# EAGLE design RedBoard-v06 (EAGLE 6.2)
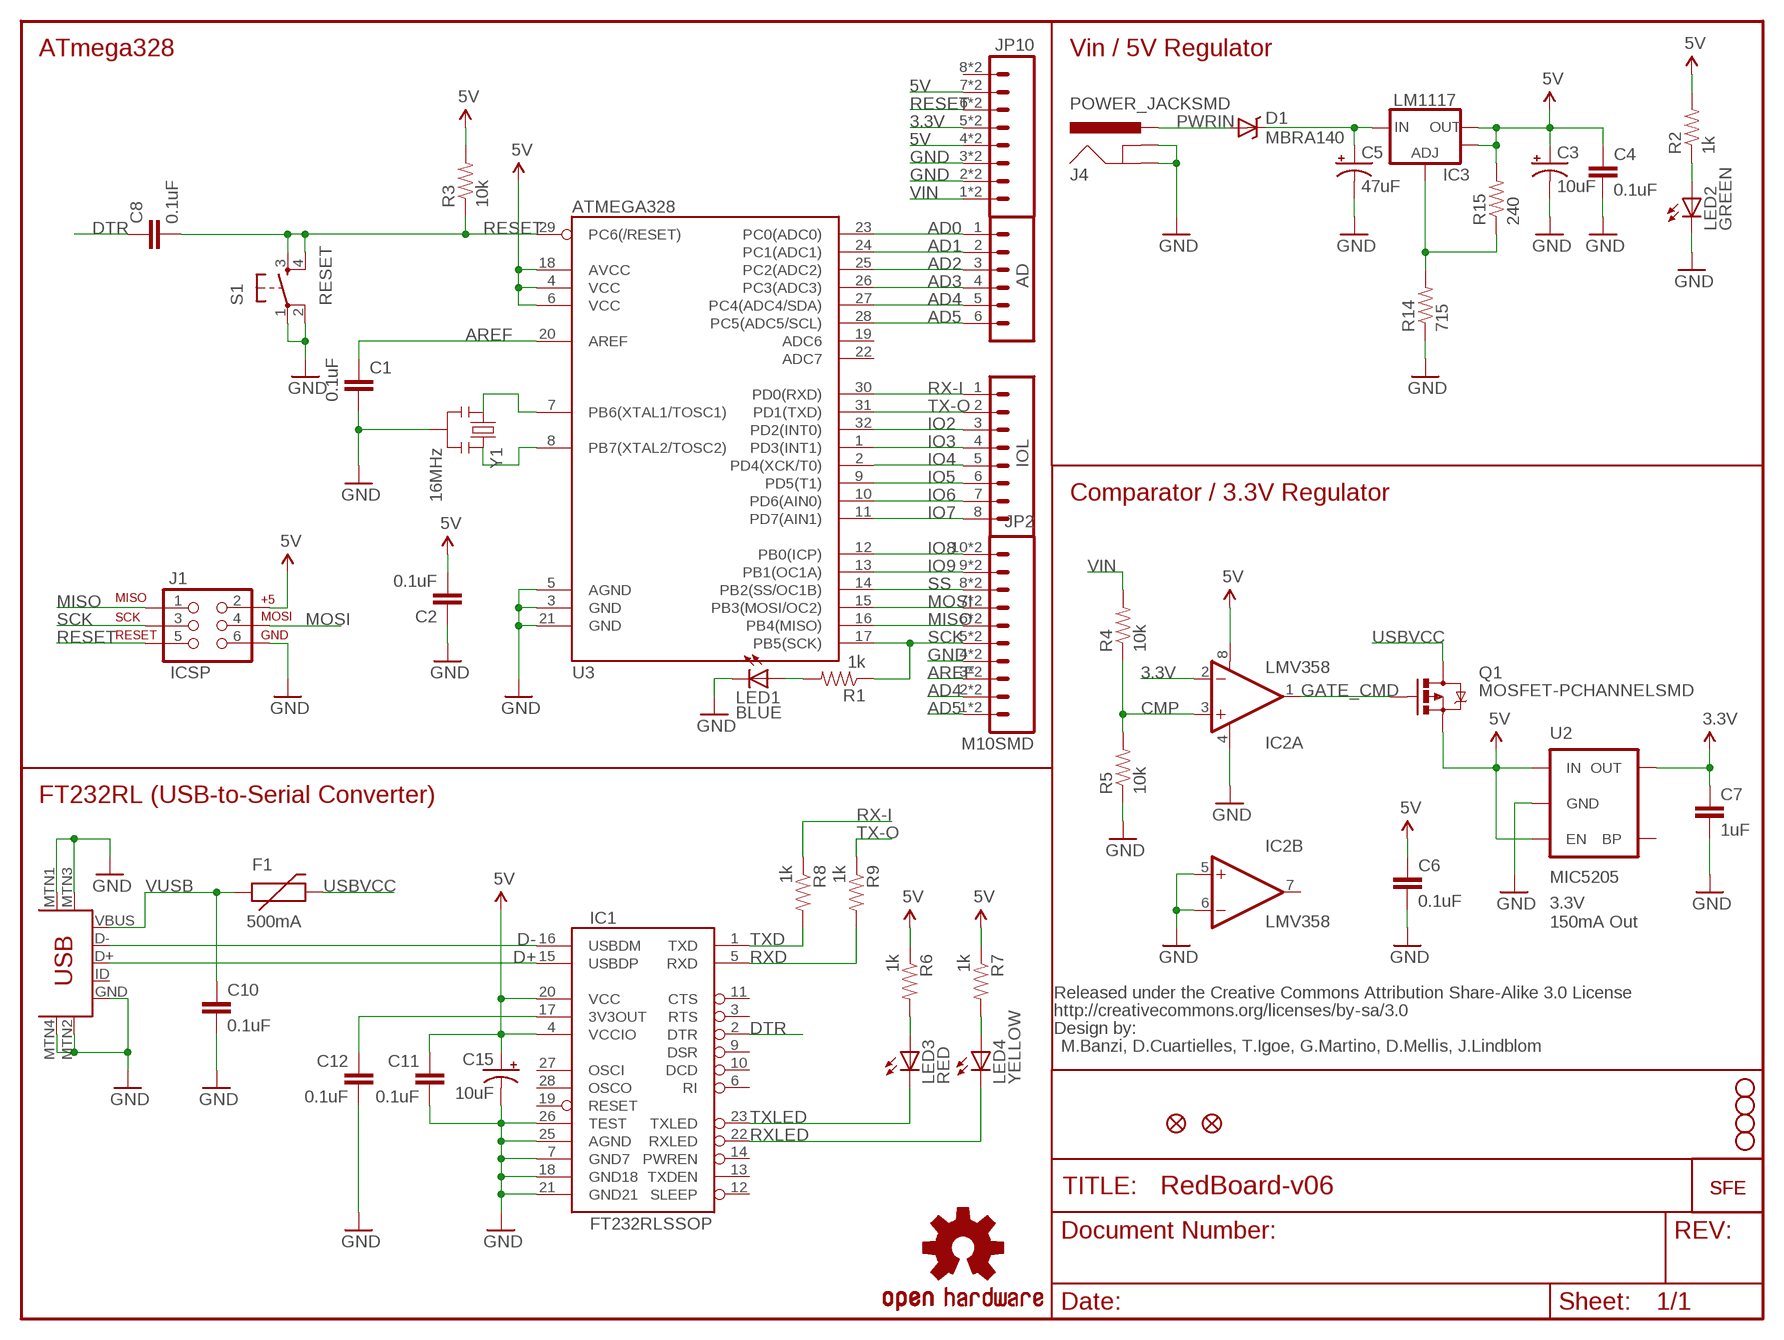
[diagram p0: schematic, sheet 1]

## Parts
AD  M06SMD-STRAIGHT-COMBO  [1X06_SMD_STRAIGHT_COMBO]
C1  0.1uF  CAP0402-CAP  [0402-CAP]
C2  0.1uF  CAP0402-CAP  [0402-CAP]
C3  10uF  CAP_POL1206  [EIA3216]
C4  0.1uF  CAP0402-CAP  [0402-CAP]
C5  47uF  CAP_POLD  [PANASONIC_D]
C6  0.1uF  CAP0402-CAP  [0402-CAP]
C7  1uF  CAP0402-CAP  [0402-CAP]
C8  0.1uF  CAP0402-CAP  [0402-CAP]
C10  0.1uF  CAP0402-CAP  [0402-CAP]
C11  0.1uF  CAP0402-CAP  [0402-CAP]
C12  0.1uF  CAP0402-CAP  [0402-CAP]
C15  10uF  CAP_POL1206  [EIA3216]
D1  MBRA140  DIODE-SCHOTTKY_  [SMA-DIODE]
F1  500mA  PTCSMD  [PTC-1206]
IC1  FT232RLSSOP  [SSOP28DB]
IC2  LMV358  OPAMP-DUALU  [SO08]
IC3  LM1117  V_REG_LM1117ALT1  [SOT223-ALT1]
IOL  M08SMD-COMBO  [1X08_SMD_COMBINED]
J1  ICSP  AVR_SPI_PRG_6PTH  [2X3]
J4  POWER_JACKSMD  [POWER_JACK_SMD]
JP1  LOGO-SFENW2  [SFE-NEW-WEB]
JP2  M10SMD  [1X10_SMD_COMBINED]
JP3  STAND-OFF  [STAND-OFF]
JP4  STAND-OFF  [STAND-OFF]
JP5  STAND-OFF  [STAND-OFF]
JP6  STAND-OFF  [STAND-OFF]
JP7  LOGO-SFESK  [SFE-LOGO-FLAME]
JP8  FIDUCIAL1X2  [FIDUCIAL-1X2]
JP9  FIDUCIAL1X2  [FIDUCIAL-1X2]
JP10  M08SMD-COMBO  [1X08_SMD_COMBINED]
LED1  BLUE  LED0603  [LED-0603]
LED2  GREEN  LED0603  [LED-0603]
LED3  RED  LED0603  [LED-0603]
LED4  YELLOW  LED0603  [LED-0603]
Q1  MOSFET-PCHANNELSMD  [SOT23-3]
R1  1k  RESISTOR0402-RES  [0402-RES]
R2  1k  RESISTOR0402-RES  [0402-RES]
R3  10k  RESISTOR0402-RES  [0402-RES]
R4  10k  RESISTOR0402-RES  [0402-RES]
R5  10k  RESISTOR0402-RES  [0402-RES]
R6  1k  RESISTOR0402-RES  [0402-RES]
R7  1k  RESISTOR0402-RES  [0402-RES]
R8  1k  RESISTOR0402-RES  [0402-RES]
R9  1k  RESISTOR0402-RES  [0402-RES]
R14  715  RESISTOR0402-RES  [0402-RES]
R15  240  RESISTOR0402-RES  [0402-RES]
S1  RESET  TAC_SWITCHSMD  [TACTILE_SWITCH_SMD]
U2  MIC5205  V_REG_LDOSMD  [SOT23-5]
U3  ATMEGA328  ATMEGA168  [TQFP32-08]
U$13  USB-MINIB-5PIN  [USB-MINIB]
U$15  CREATIVE_COMMONS  [CREATIVE_COMMONS]
U$16  OSHW-LOGOS  [OSHW-LOGO-S]
Y1  16MHz  RESONATORSMD  [RESONATOR-SMD]

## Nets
3.3V: C7.1 IC2.2(A:-IN) JP10.5 JP10.5@2 U2.5(OUT)
5V: C2.2 C3.A(+) C4.1 C6.1 C11.1 C15.A(+) IC1.4(VCCIO) IC1.20(VCC) IC2.8(A:V+) IC3.2(OUT) IC3.4(OUT) J1.2 JP10.4 JP10.4@2 JP10.7 JP10.7@2 Q1.2(S) R2.2 R3.2 R6.1 R7.1 R15.2 U2.1(IN) U2.3(EN) U3.4(VCC) U3.6(VCC) U3.18(AVCC)
AD0: AD.1 U3.23(PC0(ADC0))
AD1: AD.2 U3.24(PC1(ADC1))
AD2: AD.3 U3.25(PC2(ADC2))
AD3: AD.4 U3.26(PC3(ADC3))
AD4: AD.5 JP2.2 JP2.2@2 U3.27(PC4(ADC4/SDA))
AD5: AD.6 JP2.1 JP2.1@2 U3.28(PC5(ADC5/SCL))
AREF: C1.1 JP2.3 JP2.3@2 U3.20(AREF)
CMP: IC2.3(A:+IN) R4.1 R5.2
D+: IC1.15(USBDP) U$13.D+
D-: IC1.16(USBDM) U$13.D-
DTR: C8.1 IC1.2(DTR)
GATE_CMD: IC2.1(A:OUT) Q1.1(G)
GND: C1.2 C2.1 C3.C(-) C4.2 C5.- C6.2 C7.2 C10.2 C11.2 C12.2 C15.C(-) IC1.7(GND7) IC1.18(GND18) IC1.21(GND21) IC1.25(AGND) IC1.26(TEST) IC2.4(A:V-) IC2.5(B:+IN) IC2.6(B:-IN) J1.6 J4.GND(GNDBREAK) J4.P$4(GND) JP2.4 JP2.4@2 JP10.2 JP10.2@2 JP10.3 JP10.3@2 LED1.C LED2.C R5.1 R14.1 S1.1 S1.2 U2.2(GND) U3.3(GND) U3.5(AGND) U3.21(GND) U$13.GND U$13.MTN1(MTN2) U$13.MTN2(MTN3) U$13.MTN3(MTN1) U$13.MTN4 Y1.2
IO2: IOL.3 U3.32(PD2(INT0))
IO3: IOL.4 U3.1(PD3(INT1))
IO4: IOL.5 U3.2(PD4(XCK/T0))
IO5: IOL.6 U3.9(PD5(T1))
IO6: IOL.7 U3.10(PD6(AIN0))
IO7: IOL.8 U3.11(PD7(AIN1))
IO8: JP2.10 JP2.10@2 U3.12(PB0(ICP))
IO9: JP2.9 JP2.9@2 U3.13(PB1(OC1A))
MISO: J1.1 JP2.6 JP2.6@2 U3.16(PB4(MISO))
MOSI: J1.4 JP2.7 JP2.7@2 U3.15(PB3(MOSI/OC2))
N$1: LED1.A R1.2
N$2: LED2.A R2.1
N$3: U3.7(PB6(XTAL1/TOSC1)) Y1.1
N$4: U3.8(PB7(XTAL2/TOSC2)) Y1.3
N$5: C12.1 IC1.17(3V3OUT)
N$8: LED3.A R6.2
N$10: LED4.A R7.2
N$15: IC3.1(ADJ) R14.2 R15.1
PWRIN: D1.A J4.VIN0(PWR)
RESET: C8.2 J1.5 JP10.6 JP10.6@2 R3.1 S1.3 S1.4 U3.29(PC6(/RESET))
RX-I: IOL.1 R8.1 U3.30(PD0(RXD))
RXD: IC1.5(RXD) R9.2
RXLED: IC1.22(RXLED) LED4.C
SCK: J1.3 JP2.5 JP2.5@2 R1.1 U3.17(PB5(SCK))
SS: JP2.8 JP2.8@2 U3.14(PB2(SS/OC1B))
TX-O: IOL.2 R9.1 U3.31(PD1(TXD))
TXD: IC1.1(TXD) R8.2
TXLED: IC1.23(TXLED) LED3.C
USBVCC: F1.2 Q1.3(D)
VIN: C5.+ D1.C IC3.3(IN) JP10.1 JP10.1@2 R4.2
VUSB: C10.1 F1.1 U$13.VBUS
Unconnected: IC1.3(RTS) IC1.6(RI) IC1.9(DSR) IC1.10(DCD) IC1.11(CTS) IC1.12(SLEEP) IC1.13(TXDEN) IC1.14(PWREN) IC1.19(RESET) IC1.27(OSCI) IC1.28(OSCO) IC2.7(B:OUT) JP10.8 JP10.8@2 U2.4(BP) U3.19(ADC6) U3.22(ADC7) U$13.ID

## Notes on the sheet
- ATmega328 | Vin / 5V Regulator
- Comparator / 3.3V Regulator
- FT232RL (USB-to-Serial Converter)
- 3.3V
  150mA Out
- M.Banzi, D.Cuartielles, T.Igoe, G.Martino, D.Mellis, J.Lindblom

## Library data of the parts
AD = SparkFun:M06: Header 6 Standard 6-pin 0.1" header. Use with straight break away headers (SKU : PRT-00116), right angle break away headers (PRT-00553), swiss pins (PRT-00743), machine pins (PRT-00117), and female headers (PRT-00115). Molex polarized connector foot print use with SKU : PRT-08094 with associated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
C1 C2 C4 C6-C8 C10 C12 = SparkFun:CAP: Capacitor
C3 C5 = SparkFun:CAP_POL: Capacitor Polarized
C11 = SparkFun-Capacitors:CAP: Capacitor
C15 = SparkFun-Capacitors:CAP_POL: Capacitor Polarized
D1 = SparkFun:DIODE-SCHOTTKY
F1 = SparkFun:PTC: Resettable Fuse PTC
IC1 = SparkFun-DigitalIC:FT232RL: USB UART FT232RL 4th Generation USB UART (USB <-> Serial) Controller. Spark Fun Electronics SKU : COM-00650
IC2 = SparkFun:OPAMP-DUAL: Operational Amplifier
IC3 = Testing:V_REG_LM1117: Voltage Regulator LM1117 Standard adjustable voltage regulator but in SMD form. Spark Fun Electronics SKU : COM-00595
IOL = SparkFun:M08: Header 8 Standard 8-pin 0.1" header. Use with straight break away headers (SKU : PRT-00116), right angle break away headers (PRT-00553), swiss pins (PRT-00743), machine pins (PRT-00117), and female headers (PRT-00115).
J1 = SparkFun:AVR_SPI_PRG_6: AVR ISP 6 Pin This is the reduced ISP connector for AVR programming. Common on Arduino. This footprint will take up less PCB space and can be used with a 10-pin to 6-pin adapter such as SKU: BOB-08508
J4 = SparkFun:POWER_JACK: Power Jack This is the standard 5.5mm barrel jack for power. The PTH is the most common, proven, reliable, footprint. All others are experimental. The Slot footprint only works if the mill layer is transmitted to the PCB fab house so be warned. Spark Fun Electronics SKU : PRT-00119. Mating wall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
JP1 JP7 = SparkFun-Aesthetics:LOGO-SFE: Spark Fun Electronics PCB Logo
JP2 = SparkFun-Connectors:M10: Header 10 Standard 10-pin 0.1" header. Use with straight break away headers (SKU : PRT-00116), right angle break away headers (PRT-00553), swiss pins (PRT-00743), machine pins (PRT-00117), and female headers (PRT-00115).
JP3-JP6 = SparkFun:STAND-OFF: Stand Off
JP8 JP9 = SparkFun:FIDUCIAL: Fiducial Alignment Points
JP10 = SparkFun-Connectors:M08: Header 8 Standard 8-pin 0.1" header. Use with straight break away headers (SKU : PRT-00116), right angle break away headers (PRT-00553), swiss pins (PRT-00743), machine pins (PRT-00117), and female headers (PRT-00115).
LED1-LED4 = SparkFun:LED: LEDs
Q1 = SparkFun:MOSFET-PCHANNEL
R1-R9 R14 R15 = SparkFun:RESISTOR: Resistor
S1 = SparkFun:TAC_SWITCH: Momentary Switch Button commonly used for reset or general input. Spark Fun Electronics SKU : COM-00097
U2 = SparkFun:V_REG_LDO: Voltage Regulator LDO Standard 150mA LDO voltage regulator in SOT-23 layout. Micrel part MIC5205. BP (by-pass) pin is used to lower output noise with 470pF cap.
U3 = SparkFun:ATMEGA168
U$13 = SparkFun-Connectors:USB-MINIB: Mini-USB "B" connector with 5th pin broken out. Created new symbol breaking out 5th "ID" pin in mini/micro USB connector spec. See: http://en.wikipedia.org/wiki/Mini_usb#Cables. Uses same footprint as 4-pin symbol. Also added pins to connect to mounting / shield pads if required (probably not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
U$15 = SparkFun:CREATIVE_COMMONS
U$16 = SparkFun-Aesthetics:OSHW-LOGO: Open Source Hardware Logo This logo indicates the piece of hardware it is found on incorporates a OSHW license and/or adheres to the definition of open source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
Y1 = SparkFun-FreqCtrl:RESONATOR: Resonator Small SMD resonator. This is the itty bitty 10/20MHz resonators with built in caps. CSTCE10M0G55 and CSTCE20M0V53. Footprint has been reviewed closely but hasn't been tested yet.

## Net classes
0 default: width 0.152 mm, drill 0.305 mm, clearance 0.152 mm

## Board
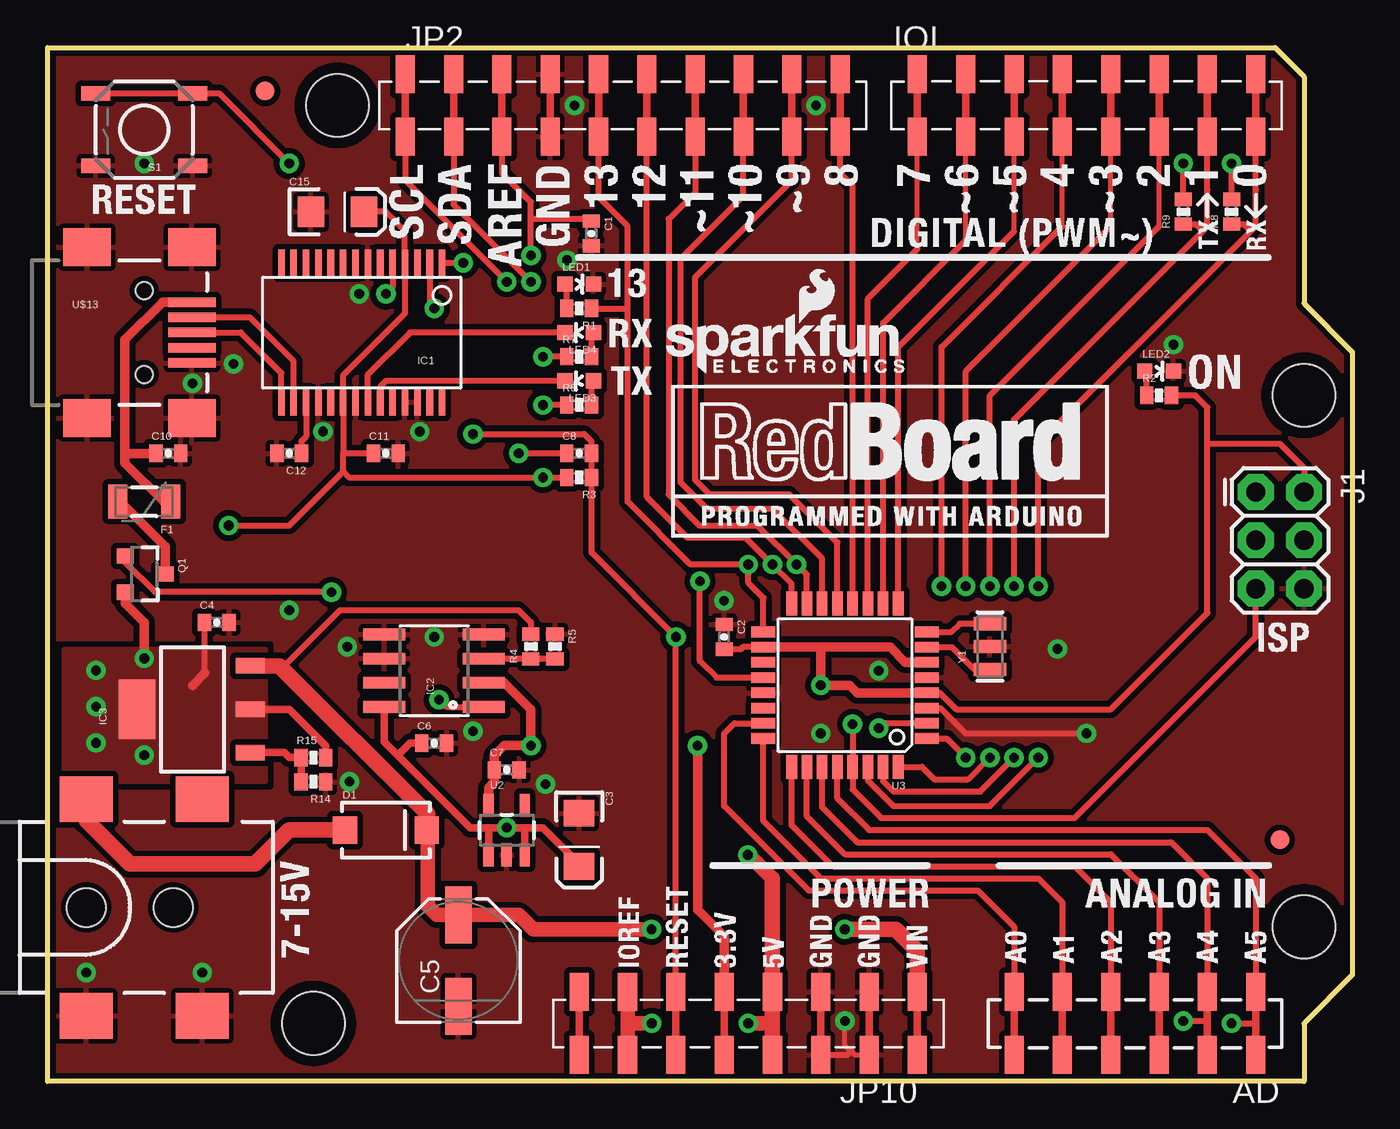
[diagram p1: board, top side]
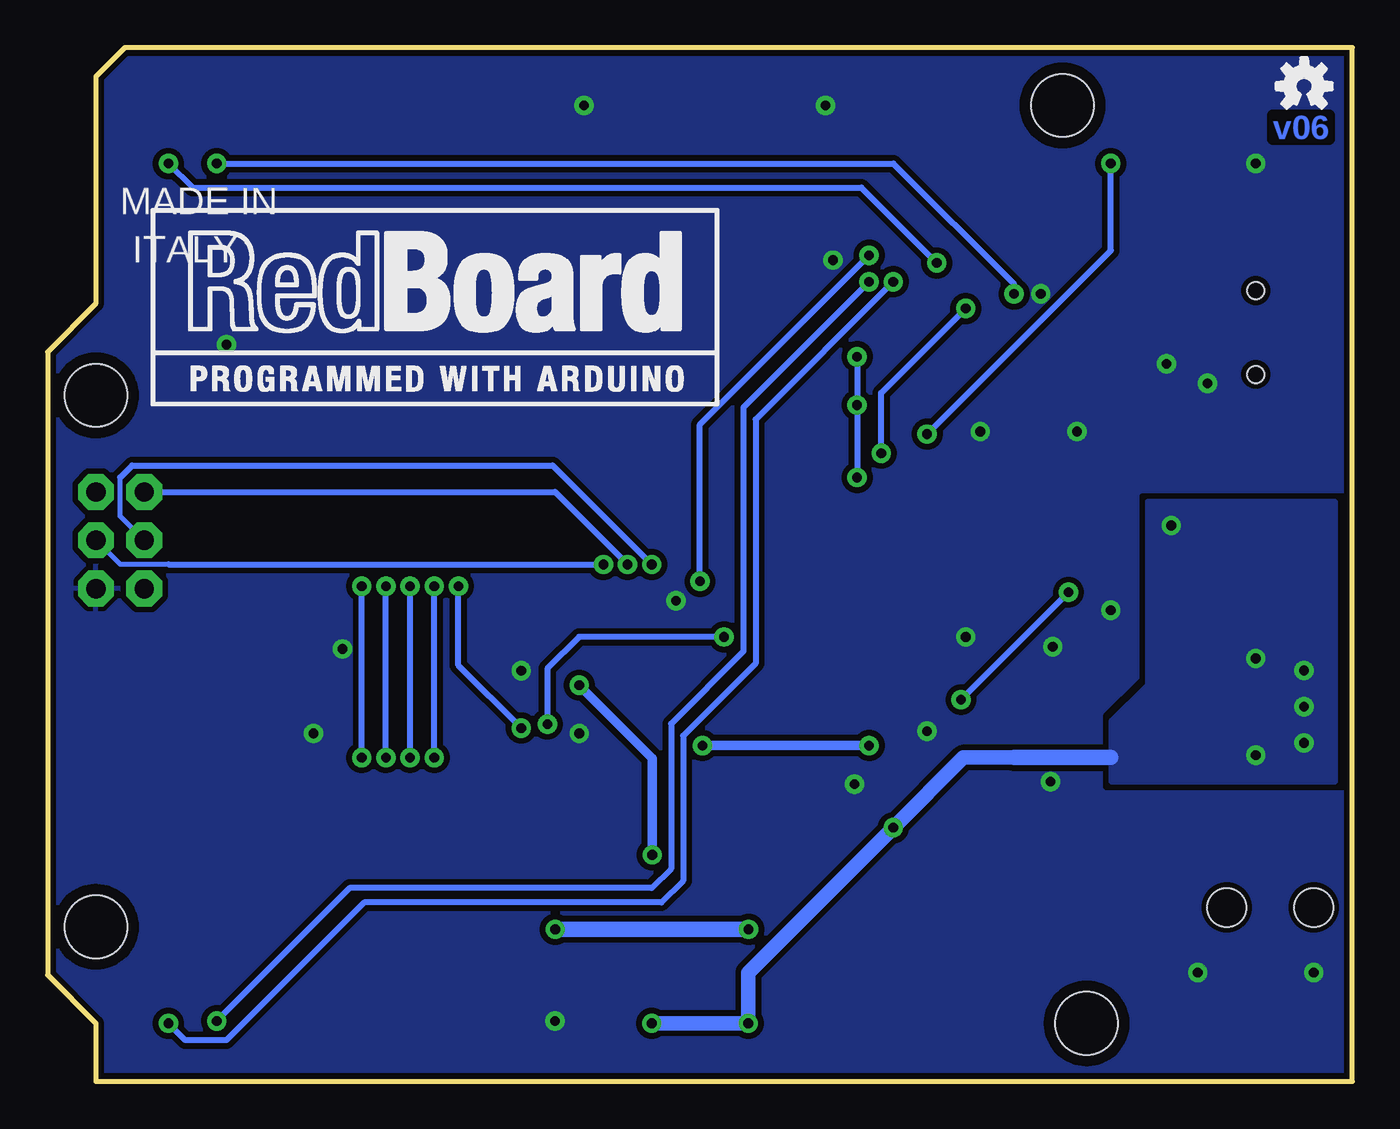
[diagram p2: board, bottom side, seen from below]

Size 68.58 x 54.36 mm. Coordinates in mm from the lower left corner, seen from the top.
Outline: 0,54.36 64.52,54.36 66.04,52.83 66.04,40.89 68.58,38.35 68.58,5.59 66.04,3.05 66.04,0 0,0 0,54.36
Copper layers (1*16): Top 0.035mm / dielectric 1.5mm / Bottom 0.035mm
Design rules: minimum track width 8mil, minimum drill 20mil, track to track 8mil, track to pad 8mil, pad to pad 8mil, via to via 8mil, smd to smd 8mil, copper to edge 8mil, drill to drill 8mil, minimum pad ring 12mil, minimum via ring 10mil, stop-mask expansion 4mil, vias tented up to drill 20mil, thermal gap 10mil
vRestrict: area 0.6,22.4 to 2,30.6; area 5.7,23.1 to 7.4,30.6; area 47.9,10.8 to 48.5,11.3; area 50.4,10.7 to 50.9,11.6; area 11.3,29.3 to 12.7,31.6; area 0.3,13 to 9.4,25

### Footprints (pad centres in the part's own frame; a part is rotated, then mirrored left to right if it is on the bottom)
1X06_SMD_STRAIGHT_COMBO = smd 1 x 2: 1 0,1.65; 1-2 0,-1.65; 2 -2.54,-1.65; 2-2 -2.54,1.65; 3 -5.08,1.65; 3-2 -5.08,-1.65; 4 -7.62,-1.65; 4-2 -7.62,1.65; 5 -10.16,1.65; 5-2 -10.16,-1.65; 6 -12.7,-1.65; 6-2 -12.7,1.65
0402-CAP = smd 0.7 x 0.9: 1 -0.65,0; 2 0.65,0
EIA3216 = smd 1.4 x 1.6: A 1.4,0; C -1.4,0
PANASONIC_D = smd 3 x 1.4: + 2.4,0; - -2.4,0
SMA-DIODE = smd 1.27 x 1.47: A -2.15,0; C 2.15,0
PTC-1206 = smd 1 x 1.8: 1 -1.4,0; 2 1.4,0
SSOP28DB = smd 0.348 x 1.397: 1 -4.225,-3.656; 2 -3.575,-3.656; 3 -2.925,-3.656; 4 -2.275,-3.656; 5 -1.625,-3.656; 6 -0.975,-3.656; 7 -0.325,-3.656; 8 0.325,-3.656; 9 0.975,-3.656; 10 1.625,-3.656; 11 2.275,-3.656; 12 2.925,-3.656; 13 3.575,-3.656; 14 4.225,-3.656; 15 4.225,3.656; 16 3.575,3.656; 17 2.925,3.656; 18 2.275,3.656; 19 1.625,3.656; 20 0.975,3.656; 21 0.325,3.656; 22 -0.325,3.656; 23 -0.975,3.656; 24 -1.625,3.656; 25 -2.275,3.656; 26 -2.925,3.656; 27 -3.575,3.656; 28 -4.225,3.656
SO08 = smd 0.61 x 2.21: 1 -1.905,-2.616; 2 -0.635,-2.616; 3 0.635,-2.616; 4 1.905,-2.616; 5 1.905,2.616; 6 0.635,2.616; 7 -0.635,2.616; 8 -1.905,2.616
SOT223-ALT1 = smd 0.813 x 1.524: 1 -2.271,-3.02; 2 0,-3.02; 3 2.288,-3.02 | smd 3.124 x 1.905: 4 0,2.921
1X08_SMD_COMBINED = smd 1 x 2: 1 0,-1.65; 1@2 0,1.65; 2 -2.54,1.65; 2@2 -2.54,-1.65; 3 -5.08,-1.65; 3@2 -5.08,1.65; 4 -7.62,1.65; 4@2 -7.62,-1.65; 5 -10.16,-1.65; 5@2 -10.16,1.65; 6 -12.7,1.65; 6@2 -12.7,-1.65; 7 -15.24,-1.65; 7@2 -15.24,1.65; 8 -17.78,1.65; 8@2 -17.78,-1.65
2X3 = drill 1.016 pad 1.88 octagon: 1 0,0; 2 0,2.54; 3 2.54,0; 4 2.54,2.54; 5 5.08,0; 6 5.08,2.54
POWER_JACK_SMD = smd 2.8 x 2.4: GND 0,-5.7; P$4 6.1,-5.7; VIN0 0,5.7; VIN1 6.1,5.7 | hole 2.032: 0,0; 4.572,0
1X10_SMD_COMBINED = smd 1 x 2: 1 0,1.65; 1@2 0,-1.65; 2 2.54,-1.65; 2@2 2.54,1.65; 3 5.08,1.65; 3@2 5.08,-1.65; 4 7.62,-1.65; 4@2 7.62,1.65; 5 10.16,1.65; 5@2 10.16,-1.65; 6 12.7,-1.65; 6@2 12.7,1.65; 7 15.24,1.65; 7@2 15.24,-1.65; 8 17.78,-1.65; 8@2 17.78,1.65; 9 20.32,1.65; 9@2 20.32,-1.65; 10 22.86,-1.65; 10@2 22.86,1.65
STAND-OFF = hole 3.302: 0,0
FIDUCIAL-1X2 = smd 1 x 1: 1 0,0
1X08_SMD_COMBINED' = smd 1 x 2: 1 0,1.65; 1@2 0,-1.65; 2 2.54,-1.65; 2@2 2.54,1.65; 3 5.08,1.65; 3@2 5.08,-1.65; 4 7.62,-1.65; 4@2 7.62,1.65; 5 10.16,1.65; 5@2 10.16,-1.65; 6 12.7,-1.65; 6@2 12.7,1.65; 7 15.24,1.65; 7@2 15.24,-1.65; 8 17.78,-1.65; 8@2 17.78,1.65
LED-0603 = smd 0.8 x 0.8: A 0,-0.75; C 0,0.75
SOT23-3 = smd 0.8 x 0.9: 1 -0.95,-1; 2 0.95,-1; 3 0,1.1
0402-RES = smd 0.7 x 0.9: 1 -0.65,0; 2 0.65,0
TACTILE_SWITCH_SMD = smd 1.524 x 0.762: 1 -2.54,1.905; 2 2.54,1.905; 3 -2.54,-1.905; 4 2.54,-1.905
SOT23-5 = smd 0.55 x 1.2: 1 -0.95,-1.3; 2 0,-1.3; 3 0.95,-1.3; 4 0.95,1.3; 5 -0.95,1.3
TQFP32-08 = smd 1.27 x 0.559: 1 -4.293,2.8; 2 -4.293,2; 3 -4.293,1.2; 4 -4.293,0.4; 5 -4.293,-0.4; 6 -4.293,-1.2; 7 -4.293,-2; 8 -4.293,-2.8; 17 4.293,-2.8; 18 4.293,-2; 19 4.293,-1.2; 20 4.293,-0.4; 21 4.293,0.4; 22 4.293,1.2; 23 4.293,2; 24 4.293,2.8 | smd 0.559 x 1.27: 9 -2.8,-4.293; 10 -2,-4.293; 11 -1.2,-4.293; 12 -0.4,-4.293; 13 0.4,-4.293; 14 1.2,-4.293; 15 2,-4.293; 16 2.8,-4.293; 25 2.8,4.293; 26 2,4.293; 27 1.2,4.293; 28 0.4,4.293; 29 -0.4,4.293; 30 -1.2,4.293; 31 -2,4.293; 32 -2.8,4.293
USB-MINIB = smd 2.5 x 0.5: D+ 2.5,0; D- 2.5,0.8; GND 2.5,-1.6; ID 2.5,-0.8; VBUS 2.5,1.6 | smd 2.5 x 2: MTN1 -3,4.5; MTN2 2.5,4.5; MTN3 -3,-4.5; MTN4 2.5,-4.5 | hole 0.9: 0,2.2; 0,-2.2
RESONATOR-SMD = smd 0.7 x 1.7: 1 -1.2,0; 2 0,0; 3 1.2,0

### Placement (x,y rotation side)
AD  50.8,3.05 180 top
C1  28.57,44.58 270 top
C2  35.56,23.37 270 top
C3  27.94,12.7 270 top
C4  8.89,24.13 0 top
C5  21.59,6.35 90 top
C6  20.32,17.78 0 top
C7  24.13,16.38 0 top
C8  27.94,33.02 0 top
C10  6.35,33.02 0 top
C11  17.78,33.02 0 top
C12  12.7,33.02 180 top
C15  15.24,45.72 0 top
D1  17.78,13.21 0 top
F1  5.08,30.48 180 top
IC1  16.51,39.37 180 top
IC2  20.32,21.59 90 top
IC3  7.62,19.56 90 top
IOL  63.5,51.31 0 top
J1  63.5,30.99 270 top
J4  2.03,9.14 0 top
JP1  32.51,37.21 0 top
JP2  18.8,51.31 0 top
JP3  13.97,3.05 0 top
JP4  66.04,8.13 0 top
JP5  66.04,36.07 0 top
JP6  15.24,51.31 0 top
JP7  39.5,39.88 0 top
JP8  64.77,12.7 0 top
JP9  11.43,52.07 0 top
JP10  [1X08_SMD_COMBINED']  45.72,3.05 180 top
LED1  27.94,41.91 270 top
LED2  58.42,37.34 270 top
LED3  27.94,36.83 90 top
LED4  27.94,39.37 90 top
Q1  5.08,26.67 270 top
R1  27.94,40.64 180 top
R2  58.42,36.07 0 top
R3  27.94,31.75 180 top
R4  25.4,22.86 90 top
R5  26.67,22.86 270 top
R6  27.94,35.56 0 top
R7  27.94,38.1 0 top
R8  62.23,45.72 90 top
R9  59.69,45.72 90 top
R14  13.97,15.75 180 top
R15  13.97,17.02 0 top
S1  5.08,50.04 180 top
U2  24.13,13.21 0 top
U3  41.91,20.83 180 top
U$13  5.08,39.37 0 top
U$15  not placed on the board
U$16  2.54,52.32 0 bottom
Y1  49.53,22.86 90 top

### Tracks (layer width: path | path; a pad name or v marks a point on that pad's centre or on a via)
3.3V  (via drill 0.51)
  Top 0.305: JP10.5 JP10.5@2
  Top 0.508: U2.5 23.18,15.43 23.48,15.73 C7.1 23.48,17.13 24,17.65 v25.4,17.65 25.4,19.56 24,20.95 IC2.2 | JP10.5@2 35.56,7.62 34.16,9.02 v34.16,17.65
  Bottom 0.508: v25.4,17.65 v34.16,17.65
5V  (via drill 0.51)
  Top 0.305: U3.18 36.54,22.83 36.43,22.72 C2.2 | U3.4 46.88,20.43 47.75,19.56 55.88,19.56 60.96,24.64 60.96,33.53 | J1.2 66.04,32.26 64.77,33.53 60.96,33.53 | 60.96,33.53 60.96,35.43 60.33,36.07 R2.2 | R7.1 v26.04,38.1 | 15.54,33.02 IC1.20 15.54,37.12 18.79,40.38 IC1.4 18.79,44.72 17.78,45.72 C15.A | C11.1 15.54,33.02 | C4.1 8.24,21.51 8.27,21.48 | JP10.4 38.1,2.54 | 15.54,32.06 15.54,33.02 | v9.53,29.22 12.7,29.22 15.54,32.06 | R3.2 v26.04,31.75 15.84,31.75 15.54,32.06 | R6.1 v26.04,35.56
  Top 0.406: U2.1 23.18,13.27 23.11,13.34 | U2.3 25.08,13.27 25.02,13.34 | R15.2 14.62,17.64 12.7,19.56 IC3.2 | IC2.8 17.7,17.86 18.41,17.14 | 18.41,17.14 22.23,13.34 23.11,13.34 | 23.11,13.34 v24.13,13.34 25.02,13.34 | C6.1 19.05,17.78 18.41,17.14 | 25.02,13.34 26.04,13.34 27.94,11.43 C3.A
  Top 0.508: U3.6 45.09,22.03 44.28,22.83 40.64,22.83 | 40.64,22.83 U3.18 | 40.64,22.83 v40.64,20.83 42.16,20.83 42.56,20.43 U3.4 | 8.27,21.48 7.62,20.83 | Q1.2 4.08,25.13 5.08,24.13 v5.08,22.24
  Top 0.762: v36.8,11.91 36.8,11.97 38.1,10.67 | v36.83,3.05 37.85,3.05 38.1,3.3 | v31.75,3.05 30.48,3.05 | 30.48,3.05 JP10.7 | JP10.7@2 30.48,3.05
  Top 0.813: 38.1,10.67 JP10.4 38.1,3.3 38.1,2.54 JP10.4@2
  Bottom 0.305: v26.04,38.1 v26.04,35.56 v26.04,31.75
  Bottom 0.508: v36.8,11.91 36.8,16.99 v40.64,20.83
  Bottom 0.762: v36.83,3.05 v31.75,3.05 31.75,5.71 v24.13,13.34 20.45,17.02 17.78,17.02
  Bottom 0.813: 17.78,17.02 12.7,17.02
  other vias: 2.54,19.7 5.08,17.16 2.54,17.79 2.54,21.6
  pour Bottom (isolate 0.305, no thermals): 0.89,30.48 10.79,30.48 10.79,20.83 12.7,18.92 12.7,15.75 0.89,15.75
  pour Top (isolate 0.305, no thermals): 0.89,15.75 0.89,22.73 11.43,22.73 11.43,15.75
AD0
  Top 0.305: U3.23 36.1,18.83 35.56,18.29 35.56,14.48 40.01,10.03 48.9,10.03 50.8,8.13 AD.1
AD1
  Top 0.305: U3.24 37.62,13.69 40.64,10.67 52.07,10.67 53.34,9.4 AD.2
AD2
  Top 0.305: U3.25 39.11,13.47 41.27,11.3 53.98,11.3 55.88,9.4 AD.3
AD3
  Top 0.305: U3.26 39.91,13.94 41.91,11.94 55.88,11.94 58.42,9.4 AD.4
AD4  (via drill 0.51)
  Top 0.254: JP2.2@2 JP2.2
  Top 0.305: U3.27 40.71,14.41 42.55,12.57 59.05,12.57 60.96,10.67 60.96,3.17 | 60.96,3.17 AD.5 | JP2.2 21.34,46.1 v25.4,42.04 | v59.69,3.17 60.96,3.17
  Bottom 0.305: v25.4,42.04 32,35.43 32,22.61 35.81,18.8 35.81,11.18 36.83,10.16 52.7,10.16 v59.69,3.17
AD5  (via drill 0.51)
  Top 0.254: JP2.1 JP2.1@2
  Top 0.305: U3.28 41.51,14.88 43.18,13.21 60.96,13.21 63.5,10.67 AD.6 63.5,3.05 v62.23,3.05 | JP2.1@2 18.8,47.37 v24.13,42.04
  Bottom 0.305: v24.13,42.04 31.37,34.8 31.37,21.97 35.18,18.16 35.18,10.54 36.32,9.4 51.94,9.4 59.18,2.16 61.34,2.16 v62.23,3.05
AREF  (via drill 0.51)
  Top 0.305: U3.20 35.16,21.23 34.29,22.1 v34.29,26.29 | JP2.3 JP2.3@2 23.88,47.75 25.4,46.23 25.4,45.34 | C1.1 28.46,45.34 25.4,45.34 | v25.4,43.43 25.4,45.34
  Bottom 0.305: v25.4,43.43 34.29,34.54 v34.29,26.29
CMP
  Top 0.305: R5.2 R4.1 25.39,22.23 IC2.3
D+
  Top 0.305: IC1.15 12.29,37.24 10.16,39.37 U$13.D+
D-
  Top 0.305: IC1.16 12.94,37.87 10.63,40.17 U$13.D-
DTR  (via drill 0.51)
  Top 0.305: IC1.2 20.09,40.88 v20.32,40.64 | C8.1 v24.77,33.02
  Bottom 0.305: v20.32,40.64 24.77,36.2 v24.77,33.02
GATE_CMD  (via drill 0.51)
  Top 0.305: IC2.1 20.95,19.68 v20.57,20.07 | Q1.1 4.08,27.29 5.65,25.72 v14.92,25.72
  Bottom 0.305: v20.57,20.07 v14.92,25.72
GND  (via drill 0.51)
  Top 0.254: JP10.2@2 42.42,1.4 42.23,1.59 41.91,1.91 v41.91,3.17
  Top 0.305: U3.3 46.92,19.63 48.26,18.29 v54.61,18.29 | JP10.3 42.04,1.4 42.23,1.59 | JP2.4@2 JP2.4
  other vias: 20.32,23.37 15.75,22.86 5.08,48.26 15.88,15.75 22.35,18.41 59.18,38.73 26.16,15.62 40.64,18.29 27.69,51.31 43.69,21.59 53.09,22.73 12.7,24.77 35.56,25.27 2.03,5.71 8.13,5.71 14.48,34.16 9.78,37.72 7.62,36.7 16.38,41.4 27.3,43.18 40.39,51.31 19.56,34.16
  pour Top (isolate 0.305, rank 2): 0,54.36 68.58,54.36 68.58,0 0,0
  pour Bottom (isolate 0.305, rank 2): 0,54.36 68.58,54.36 68.58,0 0,0
IO2  (via drill 0.51)
  Top 0.254: 58.42,44.96 IOL.3
  Top 0.305: 58.42,44.96 49.53,36.07 v49.53,26.04 | U3.32 45.95,16.54 46.61,15.88 48.39,15.88 v49.53,17.02
  Bottom 0.305: v49.53,17.02 v49.53,26.04
IO3  (via drill 0.51)
  Top 0.254: 55.88,44.96 IOL.4
  Top 0.305: 55.88,44.96 48.26,37.34 v48.26,26.04 | U3.1 47.25,18.03 v48.26,17.02
  Bottom 0.305: v48.26,17.02 v48.26,26.04
IO4  (via drill 0.51)
  Top 0.254: 53.34,44.96 IOL.5
  Top 0.305: 53.34,44.96 46.99,38.61 v46.99,26.04 | U3.2 43.94,18.83 v43.69,18.57
  Bottom 0.305: v43.69,18.57 46.99,21.88 v46.99,26.04
IO5
  Top 0.254: 50.8,44.7 IOL.6
  Top 0.305: U3.9 44.71,38.61 50.8,44.7
IO6
  Top 0.254: 48.26,44.23 IOL.7
  Top 0.305: U3.10 43.91,39.88 48.26,44.23
IO7
  Top 0.254: 45.72,43.76 IOL.8
  Top 0.305: U3.11 43.11,41.15 45.72,43.76
IO8
  Top 0.305: U3.12 42.31,47.1 41.66,47.75 JP2.10 JP2.10@2
IO9
  Top 0.305: JP2.9 JP2.9@2 39.12,47.35 34.04,42.27 34.04,31.62 34.8,30.86 38.99,30.86 41.51,28.34 U3.13
MISO  (via drill 0.51)
  Top 0.305: U3.16 39.11,26.17 v38.1,27.18 36.7,28.57 33.66,28.57 31.5,30.73 JP2.6 JP2.6@2
  Bottom 0.305: J1.1 41.91,30.99 v38.1,27.18
MOSI  (via drill 0.51)
  Top 0.305: U3.15 39.91,26.64 v39.37,27.18 37.34,29.21 34.29,29.21 32.64,30.86 32.64,45.34 34.04,46.74 JP2.7@2 JP2.7
  Bottom 0.254: 62.23,27.18 64.77,27.18 J1.4
  Bottom 0.305: 62.23,27.18 v39.37,27.18
N$1
  Top 0.305: R1.2 27.29,41.81 LED1.A
N$2
  Top 0.305: R2.1 57.77,37.24 LED2.A
N$3
  Top 0.305: U3.7 47.53,22.83 48.7,21.66 Y1.1
N$4
  Top 0.305: U3.8 47.5,23.63 47.94,24.06 Y1.3
N$5
  Top 0.305: IC1.17 13.59,33.91 13.35,33.67 C12.1
N$8
  Top 0.305: R6.2 28.59,36.73 LED3.A
N$10
  Top 0.305: R7.2 28.59,39.27 LED4.A
N$15
  Top 0.406: R14.2 R15.1 12.7,17.02 12.43,17.29 IC3.1
PWRIN
  Top 0.813: D1.A 12.7,13.21 10.92,11.43 4.32,11.43 2.03,13.72 J4.VIN0
RESET  (via drill 0.51)
  Top 0.305: J1.5 63.5,23.37 53.98,13.84 43.81,13.84 42.31,15.35 U3.29 v42.31,18.78 | S1.4 S1.3 9.02,51.94 v12.7,48.26 | JP10.6@2 JP10.6 v33.02,23.37 28.59,27.8 R3.1 C8.2 28.59,33.64 28.19,34.04 v22.35,34.04
  Bottom 0.305: v42.31,18.78 42.31,21.7 40.64,23.37 v33.02,23.37 | v22.35,34.04 12.7,43.69 v12.7,48.26
RX-I  (via drill 0.51)
  Top 0.254: 63.5,46.86 63.52,46.88
  Top 0.305: IOL.1 63.5,46.86 63.5,44.96 63.25,44.7 | U3.30 43.11,15.82 44.45,14.48 49.53,14.48 v52.07,17.02 | 63.25,44.7 52.07,33.53 v52.07,26.04 | R8.1 62.88,45.07 63.25,44.7
  Bottom 0.305: v52.07,17.02 v52.07,26.04
RXD  (via drill 0.51)
  Top 0.305: R9.2 v59.69,48.26 | IC1.5 18.14,41.76 v17.78,41.4
  Bottom 0.305: v59.69,48.26 24.13,48.26 17.78,41.91 v17.78,41.4
RXLED
  Top 0.305: IC1.22 16.84,37.16 19.05,39.37 LED4.C
SCK  (via drill 0.51)
  Top 0.305: U3.17 37.62,25.43 36.83,26.21 v36.83,27.18 33.78,27.18 30.48,30.48 30.48,40.64 | JP2.5 JP2.5@2 28.96,46.48 30.48,44.96 30.48,40.64 | R1.1 30.48,40.64
  Bottom 0.254: J1.3 64.77,29.72 64.77,31.75
  Bottom 0.305: 64.77,31.75 64.14,32.38 42.04,32.38 v36.83,27.18
SS
  Top 0.305: JP2.8@2 JP2.8 36.58,46.55 33.27,43.25 33.27,31.5 34.67,30.1 38.1,30.1 40.71,27.49 U3.14
TX-O  (via drill 0.51)
  Top 0.254: 60.96,46.86 60.95,46.88
  Top 0.305: U3.31 43.91,15.78 44.45,15.24 49.02,15.24 v50.8,17.02 | IOL.2 60.96,46.86 60.96,44.96 60.71,44.7 | v50.8,26.04 50.8,34.8 60.71,44.7 | R9.1 60.34,45.07 60.71,44.7
  Bottom 0.305: v50.8,17.02 v50.8,26.04
TXD  (via drill 0.51)
  Top 0.305: v21.84,43.03 IC1.1 | R8.2 v62.23,48.26
  Bottom 0.305: v62.23,48.26 60.96,46.99 25.81,46.99 v21.84,43.03
TXLED
  Top 0.305: LED3.C 17.78,36.83 17.48,36.53 IC1.23
USBVCC
  Top 0.508: Q1.3 6.18,28.11 3.81,30.48 F1.2
VIN  (via drill 0.51)
  Top 0.305: 12.19,21.85 12.45,21.85 15.38,24.78 24.75,24.78 25.4,24.13 R4.2 | JP10.1 JP10.1@2
  Top 0.762: v31.74,7.99 25.52,7.99 24.76,8.75 C5.+ 20.46,8.75 19.98,9.23 19.98,13.16
  Top 0.813: 19.98,13.16 D1.C 19.98,13.26 19.98,14.06 12.19,21.85 IC3.3 | v41.9,7.99 44.59,7.99 45.72,6.86 JP10.1@2
  Bottom 0.813: v31.74,7.99 v41.9,7.99
VUSB
  Top 0.508: 4.06,33.02 4.06,38.99 6.04,40.97 U$13.VBUS | 4.06,33.02 4.06,32.51 6.1,30.48 F1.1 | C10.1 4.06,33.02

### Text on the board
Bottom: v06
tNames: D.Mellis | G.Martino | T.Igoe | D.Cuartielles | M.Banzi | J.Lindblom
bNames: MADE IN | ITALY
200bmp: R
214bmp: D:/SmartProjects/Snc/a4_bn_logo2.bmp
